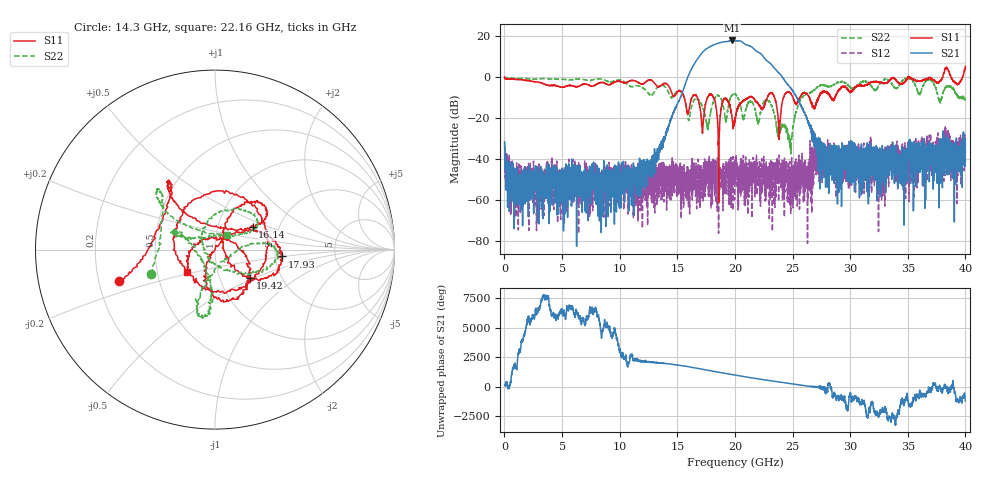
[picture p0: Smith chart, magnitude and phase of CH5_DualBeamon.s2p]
!Keysight Technologies,N5245B,MY57181321,A.14.80.03
!Date: Thursday, March 28, 2024 17:42:37
!Correction: S11(C  2-Port  )
!S21(C  2-Port  )
!S12(C  2-Port  )
!S22(C  2-Port  )
!S2P File: Measurements: S11, S21, S12, S22:
# Hz S  RI  R 50
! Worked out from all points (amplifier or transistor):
!   4000 points, 10 MHz to 40 GHz, reference 50 ohm
!   highest |S21| = 17.8 dB at 19.74 GHz (marker M1)
!   |S21| within 3 dB of that: 17.85 GHz to 21.4 GHz (3.545 GHz wide, 18.1 % of centre)
!   unconditionally stable (mu >= 1): start of sweep to 35.03 GHz; 35.17 GHz to 38.04 GHz; 38.75 GHz to 39.75 GHz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
!   at 6.67 GHz: K = 6336.76, MAG = -41.8 dB, |S12| = -48.9 dB
!   at 20.01 GHz: K = 15.27, MAG = 18.3 dB, |S12| = -48.7 dB
!   at 40 GHz: K = -1484.59, MSG = 1.4 dB, |S12| = -32.9 dB
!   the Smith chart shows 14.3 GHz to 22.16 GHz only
!   S11 on the Smith chart (normalised r, x): 14.3 GHz: 0.29, -0.15; 16.14 GHz: 1.47, +0.40; 17.93 GHz: 2.19, -0.19; 19.42 GHz: 1.39, -0.47; 22.16 GHz: 0.71, -0.18
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1e7  0.9951 -0.0383  -0.0244 0.00913  -0.00315 -0.0243  -0.9355 0.0619
6.68e9  0.4204 0.474  -0.00423 -0.00216  -0.000188 0.00182  0.857 0.1755
1.334e10  -0.4058 -0.403  -0.0115 -0.011  0.00365 -0.00459  -0.5451 -0.214
1.43e10  -0.5351 -0.1748  -0.0433 0.0531  -0.00251 0.00159  -0.3564 -0.1385
1.614e10  0.2098 0.1265  -1.061 -0.8936  0.00269 -0.00185  0.1148 0.0854
1.7e10  0.0556 0.1457  1.518 3.081  0.000512 -0.00461  0.079 0.2207
1.746e10  0.1776 -0.1489  4.4 -1.606  -0.001 0.00164  -0.0738 0.064
1.793e10  0.375 -0.0382  -1.484 -5.446  0.000109 0.000618  0.1029 -0.122
1.839e10  0.1313 0.0935  -6.428 0.5752  0.000916 -0.00485  0.3346 -0.0716
1.885e10  -0.0446 -0.1891  -0.9753 6.935  0.0007 -0.00372  0.2681 0.0391
1.942e10  0.1959 -0.1594  7.336 0.5743  0.000508 -0.00123  -0.0558 -0.1781
1.974e10  0.0969 0.0425  5.068 -5.867  0.00246 0.00622  -0.0952 -0.3414
2.001e10  -0.0851 0.0505  -0.5404 -7.528  0.00331 0.00159  -0.0652 -0.3782
2.049e10  -0.0404 -0.2207  -7.418 -0.9935  0.000886 0.00389  -0.0158 -0.1885
2.101e10  0.291 0.00715  -0.8881 5.938  0.00143 0.00197  -0.1692 0.0706
2.154e10  -0.0284 0.3122  4.882 1.589  0.00356 -0.00318  -0.2158 0.0824
2.216e10  -0.1535 -0.1242  0.7097 -3.777  0.00133 0.00504  0.0665 0.081
2.267e10  0.2446 0.0139  -2.407 -1.024  -0.00334 0.0052  0.2096 0.166
2.328e10  0.000193 0.3815  -0.8747 1.604  -0.00383 0.00377  0.1173 0.1136
2.667e10  0.1808 0.1125  0.0495 0.025  0.000443 0.000154  0.3722 0.1924
3.334e10  0.6456 -0.3907  0.00849 -0.00721  0.00208 -5.19e-05  0.3065 -0.7492
4e10  0.2927 -1.782  -0.0155 -0.0272  -0.0174 0.0145  -0.0668 0.2541
